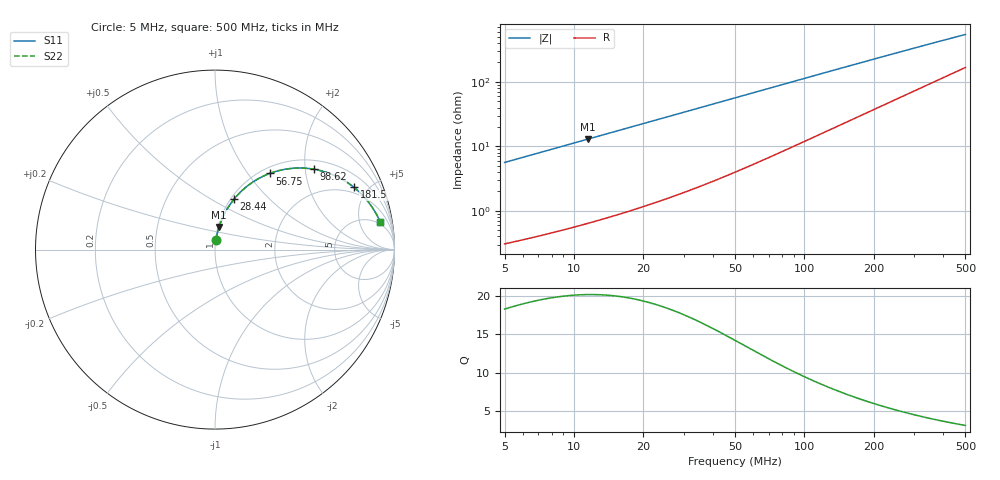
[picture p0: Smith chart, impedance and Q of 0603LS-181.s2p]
# MHz S MA R 50
!Freq  MagS11  AngS11  MagS21  AngS21  MagS12  AngS12  MagS22  AngS22
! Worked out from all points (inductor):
!   801 points, 5 MHz to 500 MHz, reference 50 ohm
!   read as one part in series: L = 179 nH near 5.116 MHz
!   highest Q = 20.2 at 11.52 MHz (marker M1), where L = 179 nH
!   S11 on the Smith chart (normalised r, x): 5 MHz: 1.01, +0.11; 28.44 MHz: 1.04, +0.64; 56.75 MHz: 1.10, +1.28; 98.62 MHz: 1.23, +2.22; 181.5 MHz: 1.63, +4.04; 500 MHz: 4, +10
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5  0.05599 83.7  0.9954 -3.2  0.9954 -3.2  0.05599 83.7
6.404275  0.07158 82.9  0.9937 -4.1  0.9937 -4.1  0.07158 82.9
7.87898  0.08788 82.1  0.9917 -5.0  0.9917 -5.0  0.08788 82.1
9.582305  0.1066 81.0  0.989 -6.1  0.989 -6.1  0.1066 81.0
11.52046  0.1277 79.8  0.9855 -7.3  0.9855 -7.3  0.1277 79.8
14.84123  0.1634 77.8  0.9785 -9.4  0.9785 -9.4  0.1634 77.8
18.79187  0.2049 75.3  0.9684 -11.8  0.9684 -11.8  0.2049 75.3
23.25252  0.2502 72.5  0.955 -14.5  0.955 -14.5  0.2502 72.5
28.44265  0.3005 69.3  0.9371 -17.5  0.9371 -17.5  0.3005 69.3
34.393  0.3548 65.8  0.914 -20.7  0.914 -20.7  0.3548 65.8
41.11213  0.4113 62.1  0.8856 -24.2  0.8856 -24.2  0.4113 62.1
56.75054  0.5229 54.3  0.8141 -31.4  0.8141 -31.4  0.5229 54.3
71.03461  0.6024 48.2  0.7486 -36.9  0.7486 -36.9  0.6024 48.2
87.89618  0.6738 42.3  0.6766 -42.1  0.6766 -42.1  0.6738 42.3
98.62114  0.7094 39.2  0.6349 -44.9  0.6349 -44.9  0.7094 39.2
131.5134  0.7857 31.6  0.528 -51.2  0.528 -51.2  0.7857 31.6
170.4002  0.8377 25.5  0.4356 -55.9  0.4356 -55.9  0.8377 25.5
181.539  0.8482 24.2  0.4143 -56.9  0.4143 -56.9  0.8482 24.2
253.4954  0.8907 17.9  0.3136 -60.9  0.3136 -60.9  0.8907 17.9
336.1012  0.9138 13.8  0.2448 -62.7  0.2448 -62.7  0.9138 13.8
418.2828  0.9262 11.2  0.2014 -63.0  0.2014 -63.0  0.9262 11.2
500  0.9337 9.4  0.1718 -62.7  0.1718 -62.7  0.9337 9.4
